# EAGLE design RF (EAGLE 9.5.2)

## Sheet 1 of 3: Board to Board Headers
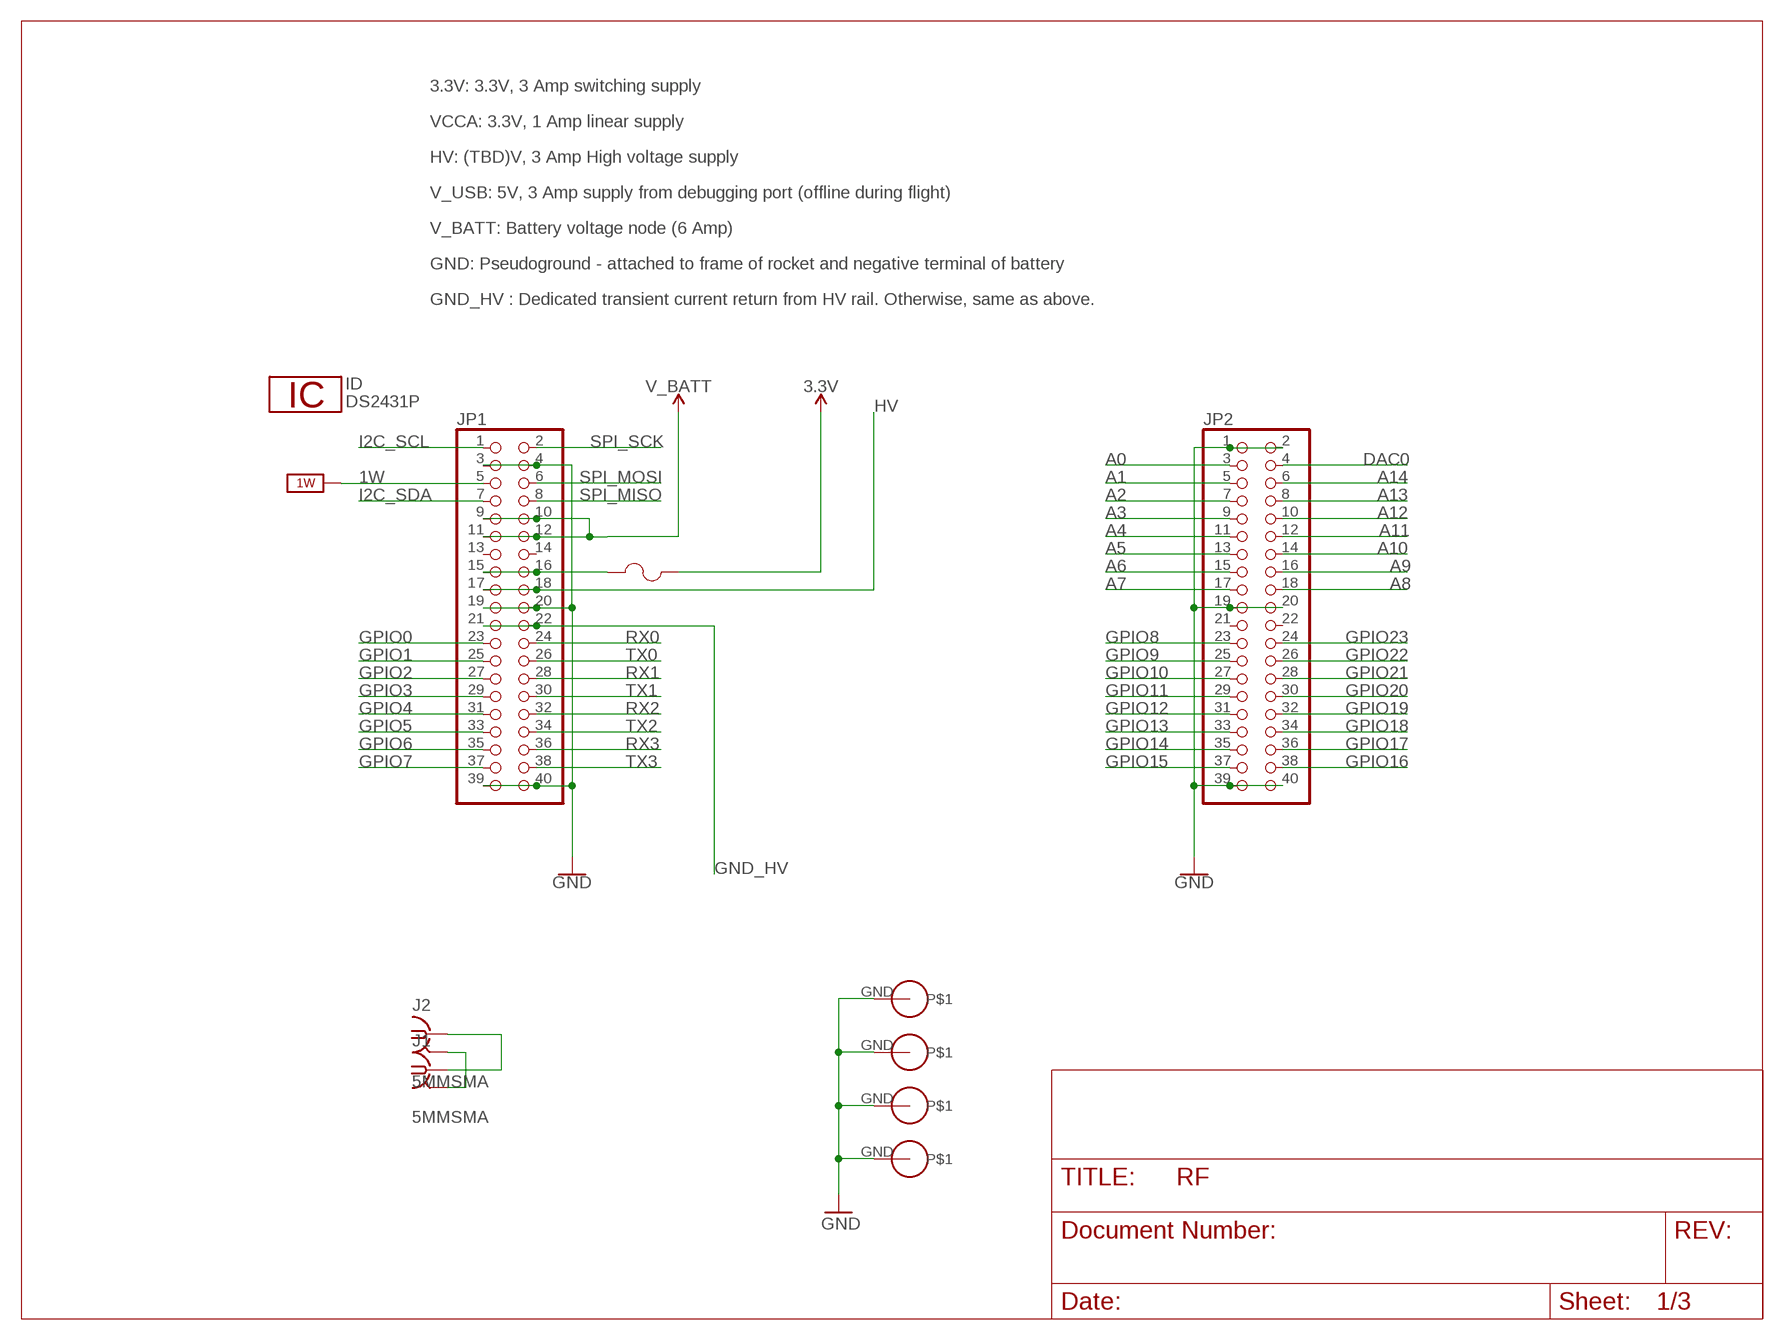
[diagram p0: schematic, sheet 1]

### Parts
F1  0603SFF150F/32-2  [FUS0603_TYCO]
ID  DS2431P  [TSOC6]
J1  5MMSMA  [5MMSMA]
J2  5MMSMA  [5MMSMA]
JP1  PINHD-2X20  [2X20]
JP2  PINHD-2X20  [2X20]
U$1  PS/104-MOUNTING-HOLE  [PC/104-MOUNTING-HOLE]
U$2  PS/104-MOUNTING-HOLE  [PC/104-MOUNTING-HOLE]
U$3  PS/104-MOUNTING-HOLE  [PC/104-MOUNTING-HOLE]
U$4  PS/104-MOUNTING-HOLE  [PC/104-MOUNTING-HOLE]

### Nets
1W: JP1.5 ; supply symbol labelled 1W_SUP
3.3V: F1.2 ; also sheet 2
A0: JP2.3
A1: JP2.5
A2: JP2.7
A3: JP2.9
A4: JP2.11
A5: JP2.13
A6: JP2.15
A7: JP2.17
A8: JP2.18
A9: JP2.16
A10: JP2.14
A11: JP2.12
A12: JP2.10
A13: JP2.8
A14: JP2.6
DAC0: JP2.4
GND: J1.GND J1.GND1 J1.GND2 J1.GND3 J2.GND J2.GND1 J2.GND2 J2.GND3 JP1.3 JP1.4 JP1.19 JP1.20 JP1.39 JP1.40 JP2.1 JP2.2 JP2.19 JP2.20 JP2.39 JP2.40 U$1.GND U$2.GND U$3.GND U$4.GND ; also sheet 2
GND_HV: JP1.21 JP1.22
GPIO0: JP1.23
GPIO1: JP1.25
GPIO2: JP1.27
GPIO3: JP1.29
GPIO4: JP1.31
GPIO5: JP1.33
GPIO6: JP1.35
GPIO7: JP1.37
GPIO8: JP2.23
GPIO9: JP2.25
GPIO10: JP2.27
GPIO11: JP2.29
GPIO12: JP2.31
GPIO13: JP2.33
GPIO14: JP2.35
GPIO15: JP2.37
GPIO16: JP2.38
GPIO17: JP2.36
GPIO18: JP2.34
GPIO19: JP2.32
GPIO20: JP2.30
GPIO21: JP2.28
GPIO22: JP2.26
GPIO23: JP2.24
HV: JP1.17 JP1.18
I2C_SCL: JP1.1
I2C_SDA: JP1.7
N$3: F1.1 JP1.15 JP1.16
N$4: JP1.9 JP1.10 JP1.11 JP1.12
N$8: J1.RF J2.RF
RX0: JP1.24 ; also sheet 2
RX1: JP1.28 ; also sheet 2
RX2: JP1.32 ; also sheet 2
RX3: JP1.36
SPI_MISO: JP1.8
SPI_MOSI: JP1.6
SPI_SCK: JP1.2
TX0: JP1.26 ; also sheet 2
TX1: JP1.30 ; also sheet 2
TX2: JP1.34 ; also sheet 2
TX3: JP1.38
Unconnected: JP1.13 JP1.14 JP2.21 JP2.22

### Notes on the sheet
- 3.3V: 3.3V, 3 Amp switching supply
- VCCA: 3.3V, 1 Amp linear supply
- HV: (TBD)V, 3 Amp High voltage supply
- V_USB: 5V, 3 Amp supply from debugging port (offline during flight)
- V_BATT: Battery voltage node (6 Amp)
- GND: Pseudoground - attached to frame of rocket and negative terminal of battery
- GND_HV : Dedicated transient current return from HV rail. Otherwise, same as above.

## Sheet 2 of 3: RN2483 434MHz RF module
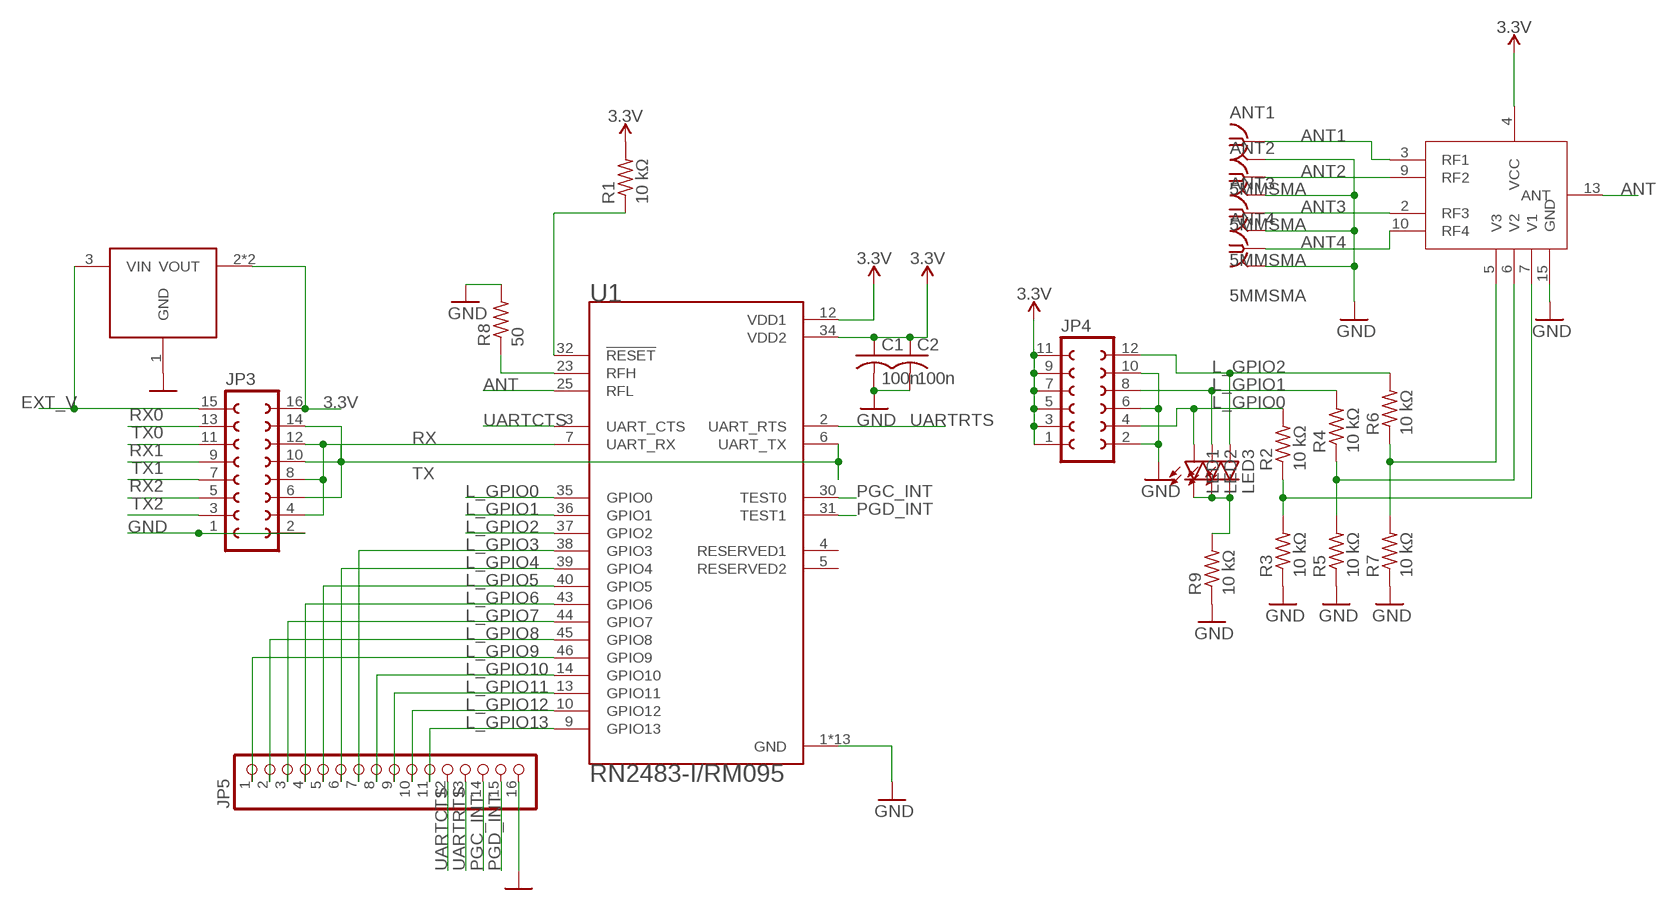
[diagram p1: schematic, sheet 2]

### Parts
ANT1  5MMSMA  [5MMSMA]
ANT2  5MMSMA  [5MMSMA]
ANT3  5MMSMA  [5MMSMA]
ANT4  5MMSMA  [5MMSMA]
C1  100n  C-USC0805  [C0805]
C2  100n  C-USC0805  [C0805]
JP3  FE08-2  [FE08-2]
JP4  FE06-2  [FE06-2]
JP5  PINHD-1X16  [1X16]
LED1  LEDSMT1206  [1206]
LED2  LEDSMT1206  [1206]
LED3  LEDSMT1206  [1206]
R1  10 kΩ  R-US_R1206  [R1206]
R2  10 kΩ  R-US_R1206  [R1206]
R3  10 kΩ  R-US_R1206  [R1206]
R4  10 kΩ  R-US_R1206  [R1206]
R5  10 kΩ  R-US_R1206  [R1206]
R6  10 kΩ  R-US_R1206  [R1206]
R7  10 kΩ  R-US_R1206  [R1206]
R8  50  R-US_R1206  [R1206]
R9  10 kΩ  R-US_R1206  [R1206]
U1  RN2483-I/RM095  [MICROCHIP_RN2483-I/RM095]
U2  SKY13414  [QFN45P200X200X55-15N]
U3  LDL1117S33R  [SOT223]

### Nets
3.3V: C1.1 C2.1 JP3.16 JP4.1 JP4.3 JP4.5 JP4.7 JP4.9 JP4.11 R1.2 U1.12(VDD1) U1.34(VDD2) U2.4(VCC) U3.2(VOUT) U3.4(VOUT) ; also sheet 1
ANT: U1.25(RFL) U2.13(ANT)
ANT1: ANT1.RF U2.3(RF1)
ANT2: ANT2.RF U2.9(RF2)
ANT3: ANT3.RF U2.2(RF3)
ANT4: ANT4.RF U2.10(RF4)
EXT_V: JP3.15 U3.3(VIN)
GND: ANT1.GND ANT1.GND1 ANT1.GND2 ANT1.GND3 ANT2.GND ANT2.GND1 ANT2.GND2 ANT2.GND3 ANT3.GND ANT3.GND1 ANT3.GND2 ANT3.GND3 ANT4.GND ANT4.GND1 ANT4.GND2 ANT4.GND3 C1.2 C2.2 JP3.1 JP3.2 JP4.2 JP4.6 JP4.10 JP5.16 R3.1 R5.1 R7.1 R8.2 R9.1 U1.1(GND) U1.8(GND) U1.11(GND) U1.20(GND) U1.21(GND) U1.22(GND) U1.24(GND) U1.26(GND) U1.27(GND) U1.28(GND) U1.33(GND) U1.41(GND) U1.47(GND) U2.15(GND) U3.1(GND) ; also sheet 1
L_GPIO0: JP4.4 LED1.A R2.2 U1.35(GPIO0)
L_GPIO1: JP4.8 LED2.A R4.2 U1.36(GPIO1)
L_GPIO2: JP4.12 LED3.A R6.2 U1.37(GPIO2)
L_GPIO3: JP5.7 U1.38(GPIO3)
L_GPIO4: JP5.6 U1.39(GPIO4)
L_GPIO5: JP5.5 U1.40(GPIO5)
L_GPIO6: JP5.4 U1.43(GPIO6)
L_GPIO7: JP5.3 U1.44(GPIO7)
L_GPIO8: JP5.2 U1.45(GPIO8)
L_GPIO9: JP5.1 U1.46(GPIO9)
L_GPIO10: JP5.8 U1.14(GPIO10)
L_GPIO11: JP5.9 U1.13(GPIO11)
L_GPIO12: JP5.10 U1.10(GPIO12)
L_GPIO13: JP5.11 U1.9(GPIO13)
N$1: R2.1 R3.2 U2.7(V1)
N$2: R4.1 R5.2 U2.6(V2)
N$5: LED1.C LED2.C LED3.C R9.2
N$7: R6.1 R7.2 U2.5(V3)
N$9: R1.1 U1.32(!RESET)
N$10: R8.1 U1.23(RFH)
PGC_INT: JP5.14 U1.30(TEST0)
PGD_INT: JP5.15 U1.31(TEST1)
RX: JP3.6 JP3.10 JP3.14 U1.6(UART_TX)
RX0: JP3.13 ; also sheet 1
RX1: JP3.9 ; also sheet 1
RX2: JP3.5 ; also sheet 1
TX: JP3.4 JP3.8 JP3.12 U1.7(UART_RX)
TX0: JP3.11 ; also sheet 1
TX1: JP3.7 ; also sheet 1
TX2: JP3.3 ; also sheet 1
UARTCTS: JP5.12 U1.3(UART_CTS)
UARTRTS: JP5.13 U1.2(UART_RTS)
Unconnected: U1.4(RESERVED1) U1.5(RESERVED2)

## Sheet 3 of 3: RN2903 903MHz RF module

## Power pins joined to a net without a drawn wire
1W: ID.2(1W)
GND: ID.1(GND)

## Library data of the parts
ANT1-ANT4 J1 J2 = CUINSPACE_Managed:5MMSMA
C1 C2 = rcl:C-US: CAPACITOR, American symbol; SPICEPREFIX: C
F1 = CU inSpace 2019 Parts:0603SFF150F/32-2; MANUFACTURER_PART_NUMBER: 0603SFF150F322; VENDOR: Littelfuse Inc
ID = 1wire:DS2431: 1024-Bit EEPROM
JP1 JP2 = pinhead:PINHD-2X20: PIN HEADER
JP3 = con-lsta:FE08-2: FEMALE HEADER; OC_FARNELL: unknown; OC_NEWARK: unknown
JP4 = con-lsta:FE06-2: FEMALE HEADER; OC_FARNELL: unknown; OC_NEWARK: unknown
JP5 = pinhead:PINHD-1X16: PIN HEADER
LED1-LED3 = led:LED: LED
R1-R9 = rcl:R-US_: RESISTOR, American symbol; SPICEPREFIX: R
U1 = RN2483-I_RM095:RN2483-I/RM095: Sub-GHz Dual Band Long Range Transceiver LoRa Module; AVAILABILITY: Unavailable; DESCRIPTION: Sub-GHz Dual Band Long Range Transceiver LoRa Module; MF: Microchip; MP: RN2483-I/RM095; PACKAGE: None; PRICE: None
U2 = CUINSPACE_Managed:SKY13414
U3 = CUINSPACE_Managed:LDL1117S33R
U$1-U$4 = CU inSpace 2019 Parts:PS/104-MOUNTING-HOLE: Mounting hole for PC/104 board.

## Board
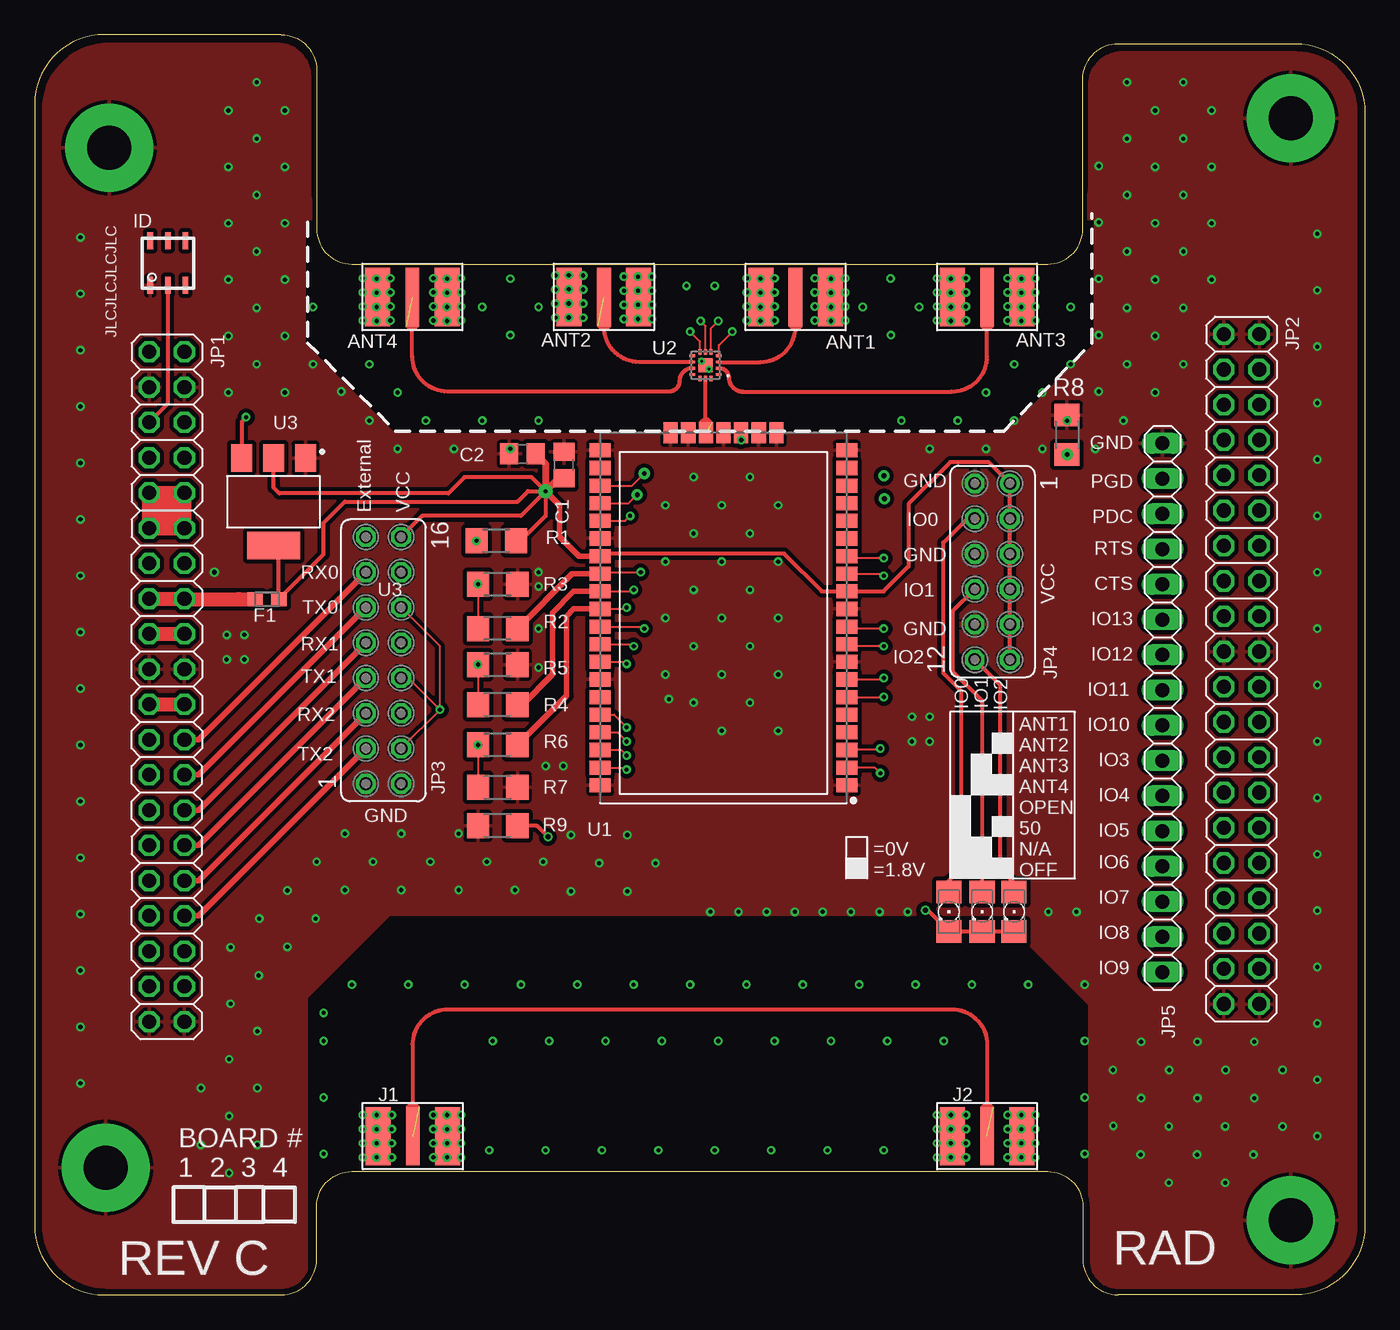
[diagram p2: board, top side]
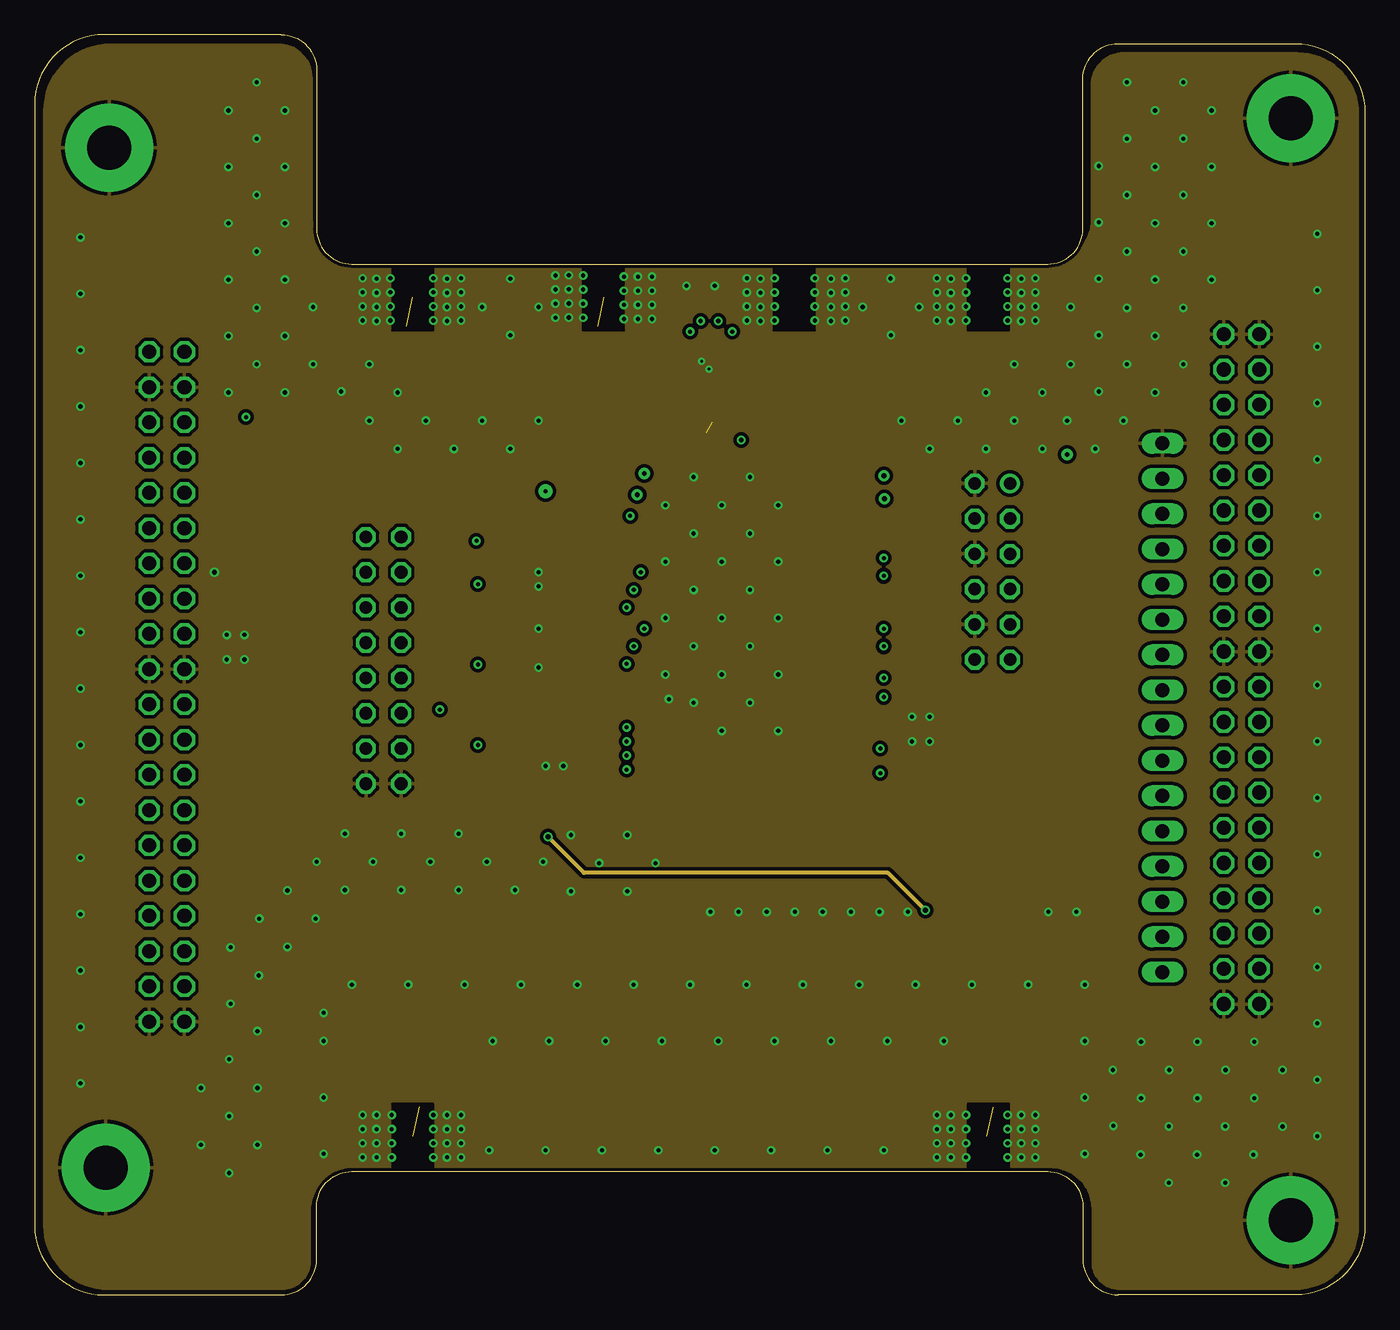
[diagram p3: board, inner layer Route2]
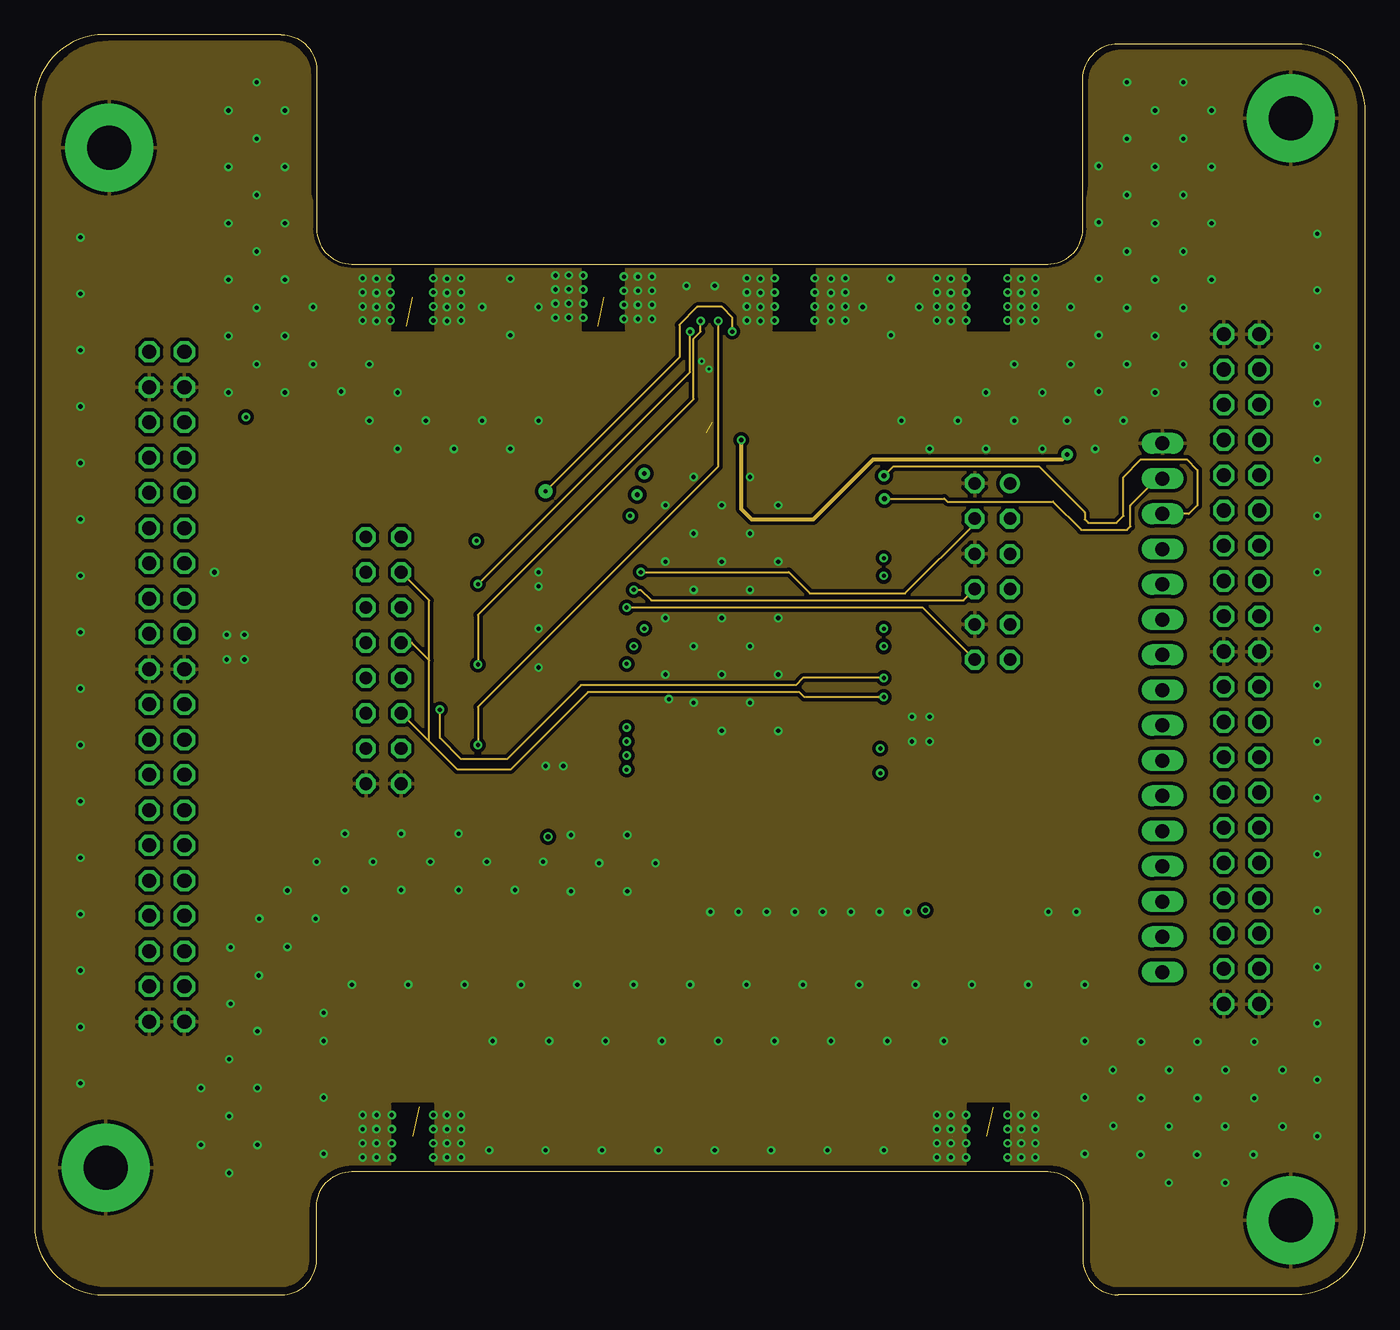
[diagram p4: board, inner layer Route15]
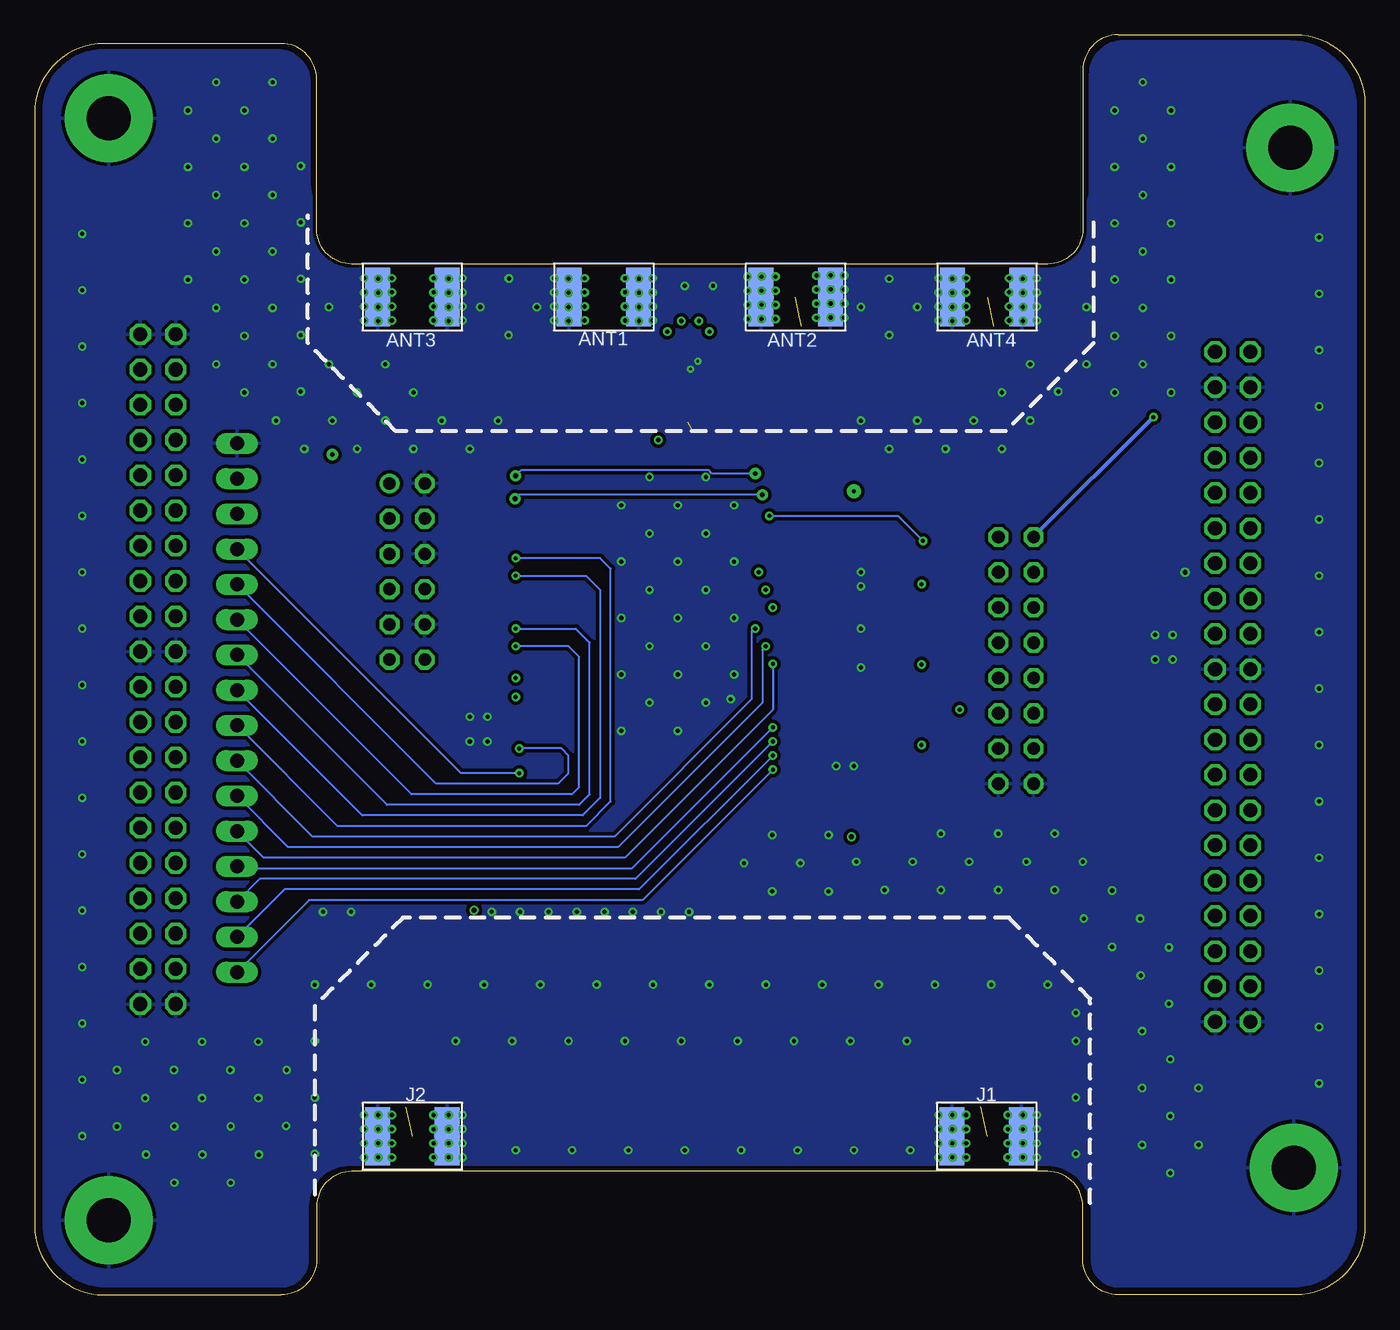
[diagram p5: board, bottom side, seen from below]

Size 95.89 x 90.81 mm. Coordinates in mm from the lower left corner, seen from the top.
Outline: 0,85.81 0,5 arc90 5,0 17.78,0 arc90 20.32,2.54 20.32,6.35 arc-90 22.86,8.89 73.03,8.89 arc-90 75.56,6.35 75.56,2.54 arc90 78.11,0 90.89,0 arc90 95.89,5 95.89,85.17 arc90 90.89,90.17 78.11,90.17 arc90 75.56,87.63 75.56,76.82 arc-90 73.03,74.28 22.86,74.28 arc-90 20.32,76.82 20.32,88.27 arc90 17.78,90.81 5,90.81 arc90 0,85.81
Copper layers (1+2*15+16): Top 0.035mm / dielectric 0.2mm / Route2 0.0175mm / dielectric 1.065mm / Route15 0.0175mm / dielectric 0.2mm / Bottom 0.035mm
Design rules "dirt_cheap_dirty_boards.v1 *": minimum track width 5mil, minimum drill 0.2mm, track to track 5mil, track to pad 5mil, pad to pad 5mil, via to via 5mil, smd to smd 0mil, copper to edge 10mil, drill to drill 10mil, minimum pad ring 10mil, minimum via ring 6mil, stop-mask expansion 2mil, vias tented up to drill 25mil, thermal gap 10mil

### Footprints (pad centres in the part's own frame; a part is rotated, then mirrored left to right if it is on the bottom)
5MMSMA = smd 1.8 x 4.2 bottom: GND 2.5,0; GND2 -2.5,0 | smd 1.8 x 4.2: GND1 -2.5,0; GND3 2.5,0 | smd 1 x 4.2: RF 0,0
C0805 = smd 1.3 x 1.5: 1 -0.95,0; 2 0.95,0
FUS0603_TYCO = smd 1.092 x 0.991: 1 -0.851,0; 2 0.851,0
TSOC6 = smd 0.406 x 1.219: 1 -1.27,-1.6; 2 0,-1.6; 3 1.27,-1.6; 4 1.27,1.6; 5 0,1.6; 6 -1.27,1.6
2X20 = drill 1.016 octagon: 1 -24.13,-1.27; 2 -24.13,1.27; 3 -21.59,-1.27; 4 -21.59,1.27; 5 -19.05,-1.27; 6 -19.05,1.27; 7 -16.51,-1.27; 8 -16.51,1.27; 9 -13.97,-1.27; 10 -13.97,1.27; 11 -11.43,-1.27; 12 -11.43,1.27; 13 -8.89,-1.27; 14 -8.89,1.27; 15 -6.35,-1.27; 16 -6.35,1.27; 17 -3.81,-1.27; 18 -3.81,1.27; 19 -1.27,-1.27; 20 -1.27,1.27; 21 1.27,-1.27; 22 1.27,1.27; 23 3.81,-1.27; 24 3.81,1.27; 25 6.35,-1.27; 26 6.35,1.27; 27 8.89,-1.27; 28 8.89,1.27; 29 11.43,-1.27; 30 11.43,1.27; 31 13.97,-1.27; 32 13.97,1.27; 33 16.51,-1.27; 34 16.51,1.27; 35 19.05,-1.27; 36 19.05,1.27; 37 21.59,-1.27; 38 21.59,1.27; 39 24.13,-1.27; 40 24.13,1.27
FE08-2 = drill 0.914 octagon: 1 -8.89,1.27; 2 -8.89,-1.27; 3 -6.35,1.27; 4 -6.35,-1.27; 5 -3.81,1.27; 6 -3.81,-1.27; 7 -1.27,1.27; 8 -1.27,-1.27; 9 1.27,1.27; 10 1.27,-1.27; 11 3.81,1.27; 12 3.81,-1.27; 13 6.35,1.27; 14 6.35,-1.27; 15 8.89,1.27; 16 8.89,-1.27
FE06-2 = drill 0.914: 1 -6.35,1.27 | drill 0.914 octagon: 2 -6.35,-1.27; 3 -3.81,1.27; 4 -3.81,-1.27; 5 -1.27,1.27; 6 -1.27,-1.27; 7 1.27,1.27; 8 1.27,-1.27; 9 3.81,1.27; 10 3.81,-1.27; 11 6.35,1.27; 12 6.35,-1.27
1X16 = drill 1.016 long: 1 -19.05,0; 2 -16.51,0; 3 -13.97,0; 4 -11.43,0; 5 -8.89,0; 6 -6.35,0; 7 -3.81,0; 8 -1.27,0; 9 1.27,0; 10 3.81,0; 11 6.35,0; 12 8.89,0; 13 11.43,0; 14 13.97,0; 15 16.51,0; 16 19.05,0
1206 = smd 1.6 x 1.803: A -1.422,0; C 1.422,0
R1206 = smd 1.6 x 1.803: 1 -1.422,0; 2 1.422,0
MICROCHIP_RN2483-I/RM095 = smd 1.524 x 1.016: 1 -8.89,12.065; 2 -8.89,10.795; 3 -8.89,9.525; 4 -8.89,8.255; 5 -8.89,6.985; 6 -8.89,5.715; 7 -8.89,4.445; 8 -8.89,3.175; 9 -8.89,1.905; 10 -8.89,0.635; 11 -8.89,-0.635; 12 -8.89,-1.905; 13 -8.89,-3.175; 14 -8.89,-4.445; 15 -8.89,-5.715; 16 -8.89,-6.985; 17 -8.89,-8.255; 18 -8.89,-9.525; 19 -8.89,-10.795; 20 -8.89,-12.065; 28 8.89,-12.065; 29 8.89,-10.795; 30 8.89,-9.525; 31 8.89,-8.255; 32 8.89,-6.985; 33 8.89,-5.715; 34 8.89,-4.445; 35 8.89,-3.175; 36 8.89,-1.905; 37 8.89,-0.635; 38 8.89,0.635; 39 8.89,1.905; 40 8.89,3.175; 41 8.89,4.445; 42 8.89,5.715; 43 8.89,6.985; 44 8.89,8.255; 45 8.89,9.525; 46 8.89,10.795; 47 8.89,12.065 | smd 1.016 x 1.524: 21 -3.81,-13.335; 22 -2.54,-13.335; 23 -1.27,-13.335; 24 0,-13.335; 25 1.27,-13.335; 26 2.54,-13.335; 27 3.81,-13.335
QFN45P200X200X55-15N = smd 0.2 x 0.395: 1 -0.675,-0.953; 2 -0.225,-0.953; 3 0.225,-0.953; 4 0.675,-0.953; 8 0.675,0.953; 9 0.225,0.953; 10 -0.225,0.953; 11 -0.675,0.953 | smd 0.395 x 0.2: 5 0.953,-0.4; 6 0.953,0; 7 0.953,0.4; 12 -0.953,0.4; 13 -0.953,0; 14 -0.953,-0.4 | smd 1 x 1: 15 0,0
SOT223 = smd 1.5 x 2: 1 -2.3,-3.15; 2 0,-3.15; 3 2.3,-3.15 | smd 3.8 x 2: 4 0,3.15
PC/104-MOUNTING-HOLE = drill 3.175 pad 6.35: GND 0,0

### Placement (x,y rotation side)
ANT1  54.85,71.9 180 top
ANT2  41.04,71.9 0 top
ANT3  68.66,71.9 0 top
ANT4  27.22,71.9 0 top
C1  38.15,59.79 90 top
C2  35.15,60.6 180 top
F1  16.75,50.13 0 top
ID  9.6,74.35 0 top
J1  27.26,11.43 0 top
J2  68.66,11.43 0 top
JP1  9.53,43.81 270 top
JP2  87,45.09 270 top
JP3  25.15,45.72 90 top
JP4  69.04,52.12 270 top
JP5  81.3,42.3 90 top
LED1  65.9,27.6 270 top
LED2  68.3,27.6 270 top
LED3  70.6,27.6 270 top
R1  33.27,54.33 0 top
R2  33.38,48.01 0 top
R3  33.38,51.21 180 top
R4  33.38,42.52 0 top
R5  33.38,45.42 180 top
R6  33.38,39.62 0 top
R7  33.38,36.58 180 top
R8  74.42,61.98 90 top
R9  33.38,33.8 0 top
U1  49.65,48.79 180 top
U2  48.36,66.99 90 top
U3  17.22,57.15 180 top
U$1  5.36,82.65 0 top
U$2  90.55,84.79 0 top
U$3  5.13,9.17 0 top
U$4  90.55,5.36 0 top

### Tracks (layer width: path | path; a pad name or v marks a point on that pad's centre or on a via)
1W
  Top 0.305: ID.2 9.6,64.21 JP1.5
3.3V  (via drill 0.3 pad 0.45, 0.3 pad 1)
  Top 0.127: U2.4 49.31,68.43 v50.29,69.41
  Top 0.305: 17.6,53.62 F1.2 20.83,53.35 20.83,55.63 22.35,57.15 34.8,57.15 35.56,57.91 v36.83,57.91 | U3.2 17.22,58.17 17.63,57.76 29.82,57.76 30.99,58.93 35.81,58.93 v36.83,57.91 | v36.83,57.91 35.05,56.13 27.94,56.13 JP3.16 | v36.83,57.91 36.83,56.13 35.11,54.42 34.78,54.42 | U1.34 40.94,53.41 54.03,53.41 56.75,50.69 U1.12 61.19,50.69 63,52.5 63,57 66,60 68.78,60 JP4.1 | JP4.11 JP4.9 JP4.7 JP4.5 JP4.3 JP4.1 | JP4.1 70.65,58.81
  Top 0.406: v36.83,57.91 37.85,56.9 37.85,54.61 39.22,53.23 U1.34 | 34.78,54.42 R1.2
  Top 0.508: C2.1 36.83,59.87 v36.83,57.91 37.76,58.84 C1.1
  Top 1.016: 17.6,53.62 U3.4
  Route15 0.127: v50.29,69.41 50.29,70.42 49.53,71.18 47.75,71.18 46.47,69.9 46.47,67.55 v36.83,57.91
ANT  (1 unrouted)
  Top 0.102: 48.84,62.88 48.54,63.18 48.24,63.18 48.04,62.98 | 48.04,62.98 47.94,62.88 48.24,62.88 48.24,63.08 48.14,62.98 | 48.14,62.98 48.04,62.98 | 48.14,62.98 48.54,62.98 48.54,63.08 48.64,62.98 | 48.64,62.98 48.74,62.88 48.54,62.88 48.64,62.98
  Top 0.293: 48.36,62.14 arc90 U1.25 48.36,62.14 | 48.36,62.14 U2.13
ANT1
  Top 0.102: 54.4,69.8 54.7,69.5 55,69.5 55.2,69.7 | 55.2,69.7 55.3,69.8 55,69.8 55,69.6 55.1,69.7 | 55.1,69.7 55.2,69.7 | 55.1,69.7 54.7,69.7 54.7,69.6 54.6,69.7 | 54.6,69.7 54.5,69.8 54.7,69.8 54.6,69.7
  Top 0.127: ANT1.RF 54.85,69.8 54.7,69.8
  Top 0.293: U2.3 52.31,67.22 arc90 54.85,69.76 ANT1.RF
ANT2  (1 unrouted)
  Top 0.102: 40.6,69.8 40.9,69.5 41.2,69.5 41.4,69.7 | 41.4,69.7 41.5,69.8 41.2,69.8 41.2,69.6 41.3,69.7 | 41.3,69.7 41.4,69.7 | 41.3,69.7 40.9,69.7 40.9,69.6 40.8,69.7 | 40.8,69.7 40.7,69.8 40.9,69.8 40.8,69.7
  Top 0.293: U2.9 43.58,67.22 arc-90 41.04,69.76 ANT2.RF
ANT3
  Top 0.102: 68.2,69.8 68.5,69.5 68.8,69.5 69,69.7 | 69,69.7 69.1,69.8 68.8,69.8 68.8,69.6 68.9,69.7 | 68.9,69.7 69,69.7 | 68.9,69.7 68.5,69.7 68.5,69.6 68.4,69.7 | 68.4,69.7 68.3,69.8 68.5,69.8 68.4,69.7
  Top 0.127: 68.5,69.8 68.66,69.8 68.66,70.5
  Top 0.293: U2.2 49.37,66.77 arc-90 50.04,66.1 arc90 51.05,65.09 66.12,65.09 arc90 68.66,67.63 68.66,70.5 ANT3.RF
ANT4  (1 unrouted)
  Top 0.102: 26.77,69.81 27.07,69.51 27.37,69.51 27.57,69.71 | 27.57,69.71 27.67,69.81 27.37,69.81 27.37,69.61 27.47,69.71 | 27.47,69.71 27.57,69.71 | 27.47,69.71 27.07,69.71 27.07,69.61 26.97,69.71 | 26.97,69.71 26.87,69.81 27.07,69.81 26.97,69.71
  Top 0.293: U2.10 U2.10 arc90 46.48,65.85 arc-90 45.72,65.09 29.76,65.09 arc-90 27.22,67.63 ANT4.RF
EXT_V  (via drill 0.3 pad 0.45)
  Top 0.305: v15.24,63.25 14.92,62.93 U3.3
  Bottom 0.305: JP3.15 v15.24,63.25
GND  (via drill 0.2 pad 0.45, 0.3 pad 0.45, 0.35)  (12 unrouted)
  Top 0.127: U2.15 48.62,66.74 v48.62,66.71
  other vias: 12.95,52.07 24.64,73.22 24.64,72.2 24.64,71.18 24.64,70.17 29.72,73.22 29.72,72.2 29.72,71.18 29.72,70.17 24.13,67.06 68.58,65.02 70.61,67.06 13.97,65.02 16,67.06 18.03,65.02 20.07,67.06 13.97,69.09 16,71.12 18.03,69.09 22.1,65.09 13.97,73.15 16,75.18 18.03,73.15 20.07,71.18 26.16,65.02 13.97,77.22 16,79.25 18.03,77.22 13.97,81.28 16,83.31 18.03,81.28 13.97,85.34 16,87.38 18.03,85.34 32.26,71.18 34.29,73.22 36.32,71.18 61.7,73.24 59.69,71.18 63.75,71.18 80.77,77.22 82.8,79.25 84.84,77.22 80.77,81.28 82.8,83.31 84.84,81.28 80.77,85.34 82.8,87.38 84.84,85.34 80.77,65.02 82.8,67.06 80.77,69.09 82.8,71.12 80.77,73.15 82.8,75.18 84.84,73.15 74.68,67.06 78.74,67.06 76.71,65.09 78.74,71.12 74.68,71.18 76.71,69.15 78.74,75.18 76.71,73.22 78.74,79.25 76.71,77.28 78.74,83.31 76.71,81.34 78.74,87.38 74.42,62.99 76.45,60.96 78.49,62.99 68.58,60.96 70.61,62.99 72.64,60.96 62.48,62.99 64.52,60.96 66.55,62.99 32.26,62.99 24.13,62.99 26.16,60.96 30.23,60.96 28.19,62.99 45.47,56.9 47.5,58.93 49.53,56.9 51.56,58.93 53.59,56.9 45.47,52.83 47.5,54.86 49.53,52.83 51.56,54.86 53.59,52.83 45.47,48.77 47.5,50.8 49.53,48.77 51.56,50.8 53.59,48.77 45.47,44.7 47.5,46.74 49.53,44.7 51.56,46.74 53.59,44.7 45.72,42.93 47.5,42.67 49.53,40.64 51.56,42.67 53.59,40.64 48.08,67.27 22.86,22.35 26.92,22.35 30.99,22.35 35.05,22.35 39.12,22.35 20.83,10.16 20.83,14.22 20.83,20.32 20.83,18.29 33.02,18.29 37.08,18.29 41.15,18.29 45.21,18.29 49.28,18.29 53.34,18.29 57.4,18.29 61.47,18.29 65.53,18.29 75.69,18.29 47.24,22.35 43.18,22.35 51.31,22.35 55.37,22.35 59.44,22.35 63.5,22.35 67.56,22.35 71.63,22.35 75.69,22.35 75.69,14.22 75.69,10.16 40.89,10.41 36.83,10.41 44.96,10.41 49.02,10.41 53.09,10.41 57.15,10.41 61.21,10.41 32.77,10.41 24.64,12.95 24.64,11.94 24.64,10.92 24.64,9.91 29.72,12.95 29.72,11.94 29.72,10.92 29.72,9.91 66.04,12.95 66.04,11.94 66.04,10.92 66.04,9.91 71.12,12.95 71.12,11.94 71.12,10.92 71.12,9.91 38.51,73.47 38.51,72.45 38.51,71.44 38.51,70.42 43.49,73.37 43.49,72.35 43.49,71.34 43.49,70.32 52.32,73.22 52.32,72.2 52.32,71.18 52.32,70.17 57.4,73.22 57.4,72.2 57.4,71.18 57.4,70.17 66.04,73.22 66.04,72.2 66.04,71.18 66.04,70.17 71.12,73.22 71.12,72.2 71.12,71.18 71.12,70.17 36.83,38.1 38.1,38.1 36.32,45.21 36.32,48.01 36.32,51.05 36.32,52.07 72.64,65.02 92.46,48.01 92.46,52.07 92.46,56.13 92.46,64.26 92.46,60.2 92.46,68.33 92.46,72.39 92.46,76.45 92.46,11.43 92.46,15.49 92.46,19.56 92.46,27.69 92.46,23.62 92.46,31.75 92.46,35.81 92.46,39.88 92.46,43.94 64.52,41.66 63.25,41.66 64.52,39.88 63.25,39.88 3.3,15.24 3.3,19.3 3.3,23.37 3.3,31.5 3.3,27.43 3.3,35.56 3.3,39.62 3.3,43.69 3.3,47.75 3.3,51.82 3.3,55.88 3.3,59.94 3.3,68.07 3.3,64.01 3.3,72.14 3.3,76.2 36.32,62.99 34.29,60.96 23.64,73.25 23.64,72.24 23.64,71.22 23.64,70.21 25.64,73.25 25.64,72.24 25.64,71.22 25.64,70.21 28.74,73.25 28.74,72.24 28.74,71.22 28.74,70.21 30.74,73.25 30.74,72.24 30.74,71.22 30.74,70.21 37.54,73.45 37.54,72.44 37.54,71.42 37.54,70.41 39.54,73.45 39.54,72.44 39.54,71.42 39.54,70.41 51.34,73.25 51.34,72.24 51.34,71.22 51.34,70.21 53.34,73.25 53.34,72.24 53.34,71.22 53.34,70.21 56.24,73.25 56.24,72.24 56.24,71.22 56.24,70.21 58.44,73.25 58.44,72.24 58.44,71.22 58.44,70.21 65.04,73.25 65.04,72.24 65.04,71.22 65.04,70.21 67.14,73.25 67.14,72.24 67.14,71.22 67.14,70.21 70.14,73.25 70.14,72.24 70.14,71.22 70.14,70.21 72.14,73.25 72.14,72.24 72.14,71.22 72.14,70.21 42.47,73.37 42.47,72.35 42.47,71.34 42.47,70.32 44.5,73.37 44.5,72.35 44.5,71.34 44.5,70.32 49.02,72.71 46.99,72.71 34.29,69.15 61.72,69.15 23.64,12.95 23.64,11.94 23.64,10.92 23.64,9.91 25.74,12.95 25.74,11.94 25.74,10.92 25.74,9.91 28.74,12.95 28.74,11.94 28.74,10.92 28.74,9.91 30.74,12.95 30.74,11.94 30.74,10.92 30.74,9.91 65.04,12.95 65.04,11.94 65.04,10.92 65.04,9.91 67.14,12.95 67.14,11.94 67.14,10.92 67.14,9.91 70.14,12.95 70.14,11.94 70.14,10.92 70.14,9.91 72.14,12.95 72.14,11.94 72.14,10.92 72.14,9.91 60.91,27.6 62.94,27.6 73.07,27.6 75.1,27.6 56.81,27.6 58.84,27.6 48.71,27.6 50.74,27.6 52.77,27.6 54.8,27.6 44.75,31.1 42.72,29.07 40.69,31.1 42.72,33.14 38.66,29.07 38.66,33.14 36.65,31.2 34.62,29.17 32.59,31.2 30.56,29.17 28.52,31.2 30.56,33.24 26.42,29.17 24.39,31.2 26.42,33.24 22.36,29.17 20.32,31.2 22.36,33.24 20.25,27.1 18.22,25.07 16.19,27.1 18.22,29.14 16.15,23 14.12,20.97 14.12,25.04 16.05,19 14.02,16.97 16.05,14.9 14.02,12.87 11.99,14.9 16.05,10.8 14.02,8.77 11.99,10.8 15.12,47.56 13.85,47.56 15.12,45.78 13.85,45.78 77.76,12.17 85.85,16.2 83.82,14.17 81.79,16.2 83.82,18.24 79.76,14.17 77.72,16.2 79.76,18.24 87.85,10.1 85.82,8.07 83.79,10.1 85.82,12.14 81.76,8.07 79.72,10.1 81.76,12.14 89.95,16.2 87.92,14.17 87.92,18.24 89.96,12.13
  pour Top (isolate 0.305, rank 3): 19.81,87.79 19.81,79.5 arc90 22.41,76.9 73.1,76.9 arc90 76.05,79.85 76.05,87.19 arc-90 78.4,89.53 90.92,89.53 arc-90 95.25,85.21 95.25,5.04 arc-90 90.72,0.51 78.11,0.51 arc-90 76.2,2.41 76.2,6.25 arc90 73.18,9.27 22.91,9.27 arc90 19.68,6.05 19.68,2.45 arc-90 17.74,0.51 5.19,0.51 arc-90 0.64,5.06 0.64,85.4 arc-90 5.4,90.17 17.43,90.17 arc-90
  pour Bottom (isolate 0.254): 19.81,87.92 19.81,79.63 arc90 22.41,77.03 73.1,77.03 arc90 76.05,79.98 76.05,87.31 arc-90 78.4,89.66 90.92,89.66 arc-90 95.25,85.33 95.25,5.17 arc-90 90.72,0.64 78.11,0.64 arc-90 76.2,2.54 76.2,6.38 arc90 73.18,9.4 22.91,9.4 arc90 19.68,6.17 19.68,2.58 arc-90 17.74,0.64 5.19,0.64 arc-90 0.64,5.19 0.64,85.53 arc-90 5.4,90.3 17.43,90.3 arc-90
  pour Route15 (isolate 0.254): 19.81,87.92 19.81,79.63 arc90 22.41,77.03 73.1,77.03 arc90 76.05,79.98 76.05,87.31 arc-90 78.4,89.66 90.92,89.66 arc-90 95.25,85.33 95.25,5.17 arc-90 90.72,0.64 78.11,0.64 arc-90 76.2,2.54 76.2,6.38 arc90 73.18,9.4 22.91,9.4 arc90 19.68,6.17 19.68,2.58 arc-90 17.74,0.64 5.19,0.64 arc-90 0.64,5.19 0.64,85.53 arc-90 5.4,90.3 17.43,90.3 arc-90
  pour Route2 (isolate 0.254): 19.91,87.72 19.91,77.93 arc90 23.71,74.13 72.8,74.13 arc90 76.25,77.58 76.25,87.21 arc-90 78.5,89.46 91.02,89.46 arc-90 95.35,85.13 95.35,4.97 arc-90 90.82,0.43 78.2,0.43 arc-90 76.3,2.34 76.3,6.18 arc90 73.28,9.2 23.01,9.2 arc90 19.79,5.97 19.79,2.38 arc-90 17.84,0.43 5.29,0.43 arc-90 0.73,4.99 0.73,85.33 arc-90 5.5,90.1 17.53,90.1 arc-90
  cutout Route15: 25.75,74.25 25.75,69.5 28.75,69.5 28.75,74.25
GND1
  cutout Route2: 25.75,74.25 25.75,69.5 28.75,69.5 28.75,74.25
GND2
  cutout Bottom: 25.75,74.25 25.75,69.5 28.75,69.5 28.75,74.25
GND6
  cutout Route15: 39.5,74.25 39.5,69.5 42.5,69.5 42.5,74.25
GND7
  cutout Route2: 39.5,74.25 39.5,69.5 42.5,69.5 42.5,74.25
GND8
  cutout Bottom: 39.5,74.25 39.5,69.5 42.5,69.5 42.5,74.25
GND9
  cutout Route15: 53.25,74.25 53.25,69.5 56.25,69.5 56.25,74.25
GND10
  cutout Route2: 53.25,74.25 53.25,69.5 56.25,69.5 56.25,74.25
GND11
  cutout Bottom: 53.25,74.25 53.25,69.5 56.25,69.5 56.25,74.25
GND12
  cutout Route15: 67.25,74.25 67.25,69.5 70.25,69.5 70.25,74.25
GND13
  cutout Route2: 67.25,74.25 67.25,69.5 70.25,69.5 70.25,74.25
GND14
  cutout Bottom: 67.25,74.25 67.25,69.5 70.25,69.5 70.25,74.25
GND15
  cutout Route15: 67.25,13.75 67.25,9 70.25,9 70.25,13.75
GND16
  cutout Route2: 67.25,13.75 67.25,9 70.25,9 70.25,13.75
GND17
  cutout Bottom: 67.25,13.75 67.25,9 70.25,9 70.25,13.75
GND18
  cutout Route15: 25.75,13.75 25.75,9 28.75,9 28.75,13.75
GND19
  cutout Route2: 25.75,13.75 25.75,9 28.75,9 28.75,13.75
GND20
  cutout Bottom: 25.75,13.75 25.75,9 28.75,9 28.75,13.75
GND_HV
  Top 1.016: JP1.21 JP1.22
HV
  Top 1.016: JP1.17 JP1.18
KEEPOUT
  cutout Top (no thermals): 19.68,77.28 19.68,68.58 26.04,62.23 69.85,62.23 76.2,68.58 76.2,77.28 75.56,77.28
KEEPOUT1
  cutout Top (no thermals): 75.82,-0.64 75.82,20.83 69.47,27.18 25.65,27.18 19.81,21.34 19.81,-0.64
L_GPIO0  (via drill 0.3 pad 0.45)
  Top 0.127: U1.35 40.87,52.07 v43.69,52.07
  Top 0.305: LED1.A 65.9,29.82 66.8,30.72 66.8,43.5 65.5,44.8 65.5,54.2 67.23,55.93 JP4.4
  Top 0.406: R2.2 38.75,51.96 U1.35
  Route15 0.127: v43.69,52.07 54.36,52.07 55.88,50.55 62.74,50.55 67.77,55.58 JP4.4
L_GPIO1  (via drill 0.3 pad 0.45)
  Top 0.127: U1.36 43.07,50.69 v43.18,50.8
  Top 0.305: JP4.8 66.2,49.28 66.2,44.9 68.3,42.8 LED2.A
  Top 0.406: U1.36 38.86,50.69 37.34,49.17 37.34,44.7 35.15,42.52 R4.2
  Route15 0.127: v43.18,50.8 43.69,50.8 44.45,50.04 66.95,50.04 JP4.8
L_GPIO2  (via drill 0.3 pad 0.45)
  Top 0.127: U1.37 42.56,49.42 v42.67,49.53
  Top 0.305: LED3.A 70.6,29.7 69.6,30.7 69.6,43.94 JP4.12
  Top 0.406: U1.37 38.86,49.42 38.35,48.91 38.35,43.18 R6.2
  Route15 0.127: JP4.12 64.01,49.53 v42.67,49.53
L_GPIO3  (via drill 0.3 pad 0.45)
  Top 0.127: U1.38 43.8,48.15 v43.94,48.01
  Bottom 0.127: v43.94,48.01 44.2,47.75 44.2,42.93 54.1,33.02 75.83,33.02 JP5.7
L_GPIO4  (via drill 0.3 pad 0.45)
  Top 0.127: U1.39 43.03,46.88 v43.18,46.74
  Bottom 0.127: v43.18,46.74 43.43,46.48 43.43,42.67 53.85,32.26 77.61,32.26 JP5.6
L_GPIO5  (via drill 0.3 pad 0.45)
  Top 0.127: U1.40 42.53,45.61 v42.67,45.47
  Bottom 0.127: v42.67,45.47 42.67,42.16 53.34,31.5 79.39,31.5 JP5.5
L_GPIO6  (via drill 0.3 pad 0.45)
  Top 0.127: U1.43 41.76,41.8 v42.67,40.89
  Bottom 0.127: v42.67,40.89 52.83,30.73 81.16,30.73 JP5.4
L_GPIO7  (via drill 0.3 pad 0.45)
  Top 0.127: U1.44 42.02,40.53 v42.67,39.88
  Bottom 0.127: v42.67,39.88 52.58,29.97 79.66,29.97 JP5.3
L_GPIO8  (via drill 0.3 pad 0.45)
  Top 0.127: U1.45 42.27,39.26 v42.67,38.86
  Bottom 0.127: v42.67,38.86 52.32,29.21 77.88,29.21 JP5.2
L_GPIO9  (via drill 0.3 pad 0.45)
  Top 0.127: U1.46 42.53,37.99 v42.67,37.85
  Bottom 0.127: v42.67,37.85 52.07,28.45 76.1,28.45 JP5.1
L_GPIO10  (via drill 0.3 pad 0.45)
  Top 0.127: v61.21,53.09 58.69,53.09 U1.14
  Bottom 0.127: v61.21,53.09 55.12,53.09 54.36,52.32 54.36,35.56 56.13,33.78 74.05,33.78 JP5.8
L_GPIO11  (via drill 0.3 pad 0.45)
  Top 0.127: U1.13 61.07,51.96 v61.21,51.82
  Bottom 0.127: v61.21,51.82 56.13,51.82 55.12,50.8 55.12,35.81 56.39,34.54 72.27,34.54 JP5.9
L_GPIO12  (via drill 0.3 pad 0.45)
  Top 0.127: v61.21,48.01 58.69,48.01 U1.10
  Bottom 0.127: v61.21,48.01 56.9,48.01 55.88,46.99 55.88,36.07 56.64,35.31 70.5,35.31 JP5.10
L_GPIO13  (via drill 0.3 pad 0.45)
  Top 0.127: v61.21,46.74 58.69,46.74 U1.9
  Bottom 0.127: v61.21,46.74 57.4,46.74 56.64,45.97 56.64,36.58 57.15,36.07 68.72,36.07 JP5.11
N$1  (via drill 0.3 pad 0.45)
  Top 0.127: U2.7 47.96,68.69 v47.24,69.41 | R3.2 R2.1
  Route15 0.127: R3.2 47.24,66.5 v47.24,69.41
  other vias: 31.95,51.21
N$2  (via drill 0.3 pad 0.45)
  Top 0.127: U2.6 48.36,69.81 v48.01,70.17 | R5.2 R4.1
  Route15 0.127: R5.2 31.95,49 47.5,64.55 47.5,68.9 48.01,69.41 v48.01,70.17
  other vias: 31.95,45.42
N$3
  Top 1.016: JP1.15 JP1.16 10.79,50.13 14.73,50.13 F1.1
N$4
  Top 1.016: 9,55.24 JP1.11 JP1.9 | 9,55.24 10,55.24 | 10,55.24 JP1.12 JP1.10 10,57.78 | JP1.9 10,57.78 | JP1.9 9,57.78 9,55.24 | 10,55.24 10,57.78
N$5  (via drill 0.35)
  Top 0.305: LED3.C LED2.C LED1.C 64.38,27.7 v64.2,27.7 | v37,33 36.2,33.8 R9.2
  Route2 0.305: v64.2,27.7 61.5,30.4 39.6,30.4 v37,33
N$7  (via drill 0.3 pad 0.45)
  Top 0.127: U2.5 48.76,69.65 v49.28,70.17 | R6.1 R7.2
  Route15 0.127: R6.1 31.95,42.37 49.28,59.69 v49.28,70.17
  other vias: 31.95,39.62
N$8  (2 unrouted)
  Top 0.102: 27.71,13.55 27.41,13.85 27.11,13.85 26.91,13.65 | 26.91,13.65 26.81,13.55 27.11,13.55 27.11,13.75 27.01,13.65 | 27.01,13.65 26.91,13.65 | 27.01,13.65 27.41,13.65 27.41,13.75 27.51,13.65 | 27.51,13.65 27.61,13.55 27.41,13.55 27.51,13.65 | 69.11,13.53 68.81,13.83 68.51,13.83 68.31,13.63 | 68.31,13.63 68.21,13.53 68.51,13.53 68.51,13.73 68.41,13.63 | 68.41,13.63 68.31,13.63 | 68.41,13.63 68.81,13.63 68.81,13.73 68.91,13.63 | 68.91,13.63 69.01,13.53 68.81,13.53 68.91,13.63
  Top 0.293: J1.RF 27.26,18.03 arc-90 29.8,20.57 66.12,20.57 arc-90 68.66,18.03 J2.RF
N$9  (via drill 0.3 pad 0.45)
  Top 0.127: U1.32 42.16,55.77 42.56,55.77 v42.93,56.13
  Bottom 0.127: v42.93,56.13 33.66,56.13 R1.1
  other vias: 31.85,54.33
N$10  (via drill 0.3 pad 0.45, 0.35 pad 0.8)
  Top 0.293: U1.23 v50.92,61.6 v50.93,61.59
  Route15 0.293: v50.93,61.59 50.93,56.64 51.69,55.88 56.13,55.88 60.45,60.2 74.07,60.2 R8.1
  other vias: 74.42,60.55
PGC_INT  (via drill 0.35 pad 0.8)
  Top 0.127: U1.30 43.07,58.31 v43.94,59.18
  Route15 0.127: v61.21,59.02 61.89,59.69 72.39,59.69 75.69,56.39 75.69,55.88 75.95,55.63 77.98,55.63 78.49,56.13 78.49,58.93 79.76,60.2 83.06,60.2 83.82,59.44 83.82,56.9 83.19,56.27 JP5.14
  Bottom 0.127: v43.94,59.18 47.05,59.18 47.29,59.42 60.81,59.42 v61.21,59.02
PGD_INT  (via drill 0.35 pad 0.8)
  Top 0.127: U1.31 42.82,57.04 v43.43,57.66
  Route15 0.127: v61.25,57.37 65.56,57.37 65.79,57.15 73.41,57.15 75.44,55.12 78.74,55.12 78.99,55.37 78.99,56.9 80.91,58.81 JP5.15
  Bottom 0.127: v43.43,57.66 60.96,57.66 v61.25,57.37
RX  (via drill 0.3 pad 0.45)
  Top 0.127: U1.6 v61.21,43.07
  Route15 0.127: v61.21,43.07 55.48,43.07 55.12,43.43 39.88,43.43 34.29,37.85 30.48,37.85 28.45,39.88 | 28.45,39.88 JP3.6 | 28.45,39.88 28.45,45.72 | 28.45,45.72 27.18,46.99 JP3.10 | 28.45,45.72 28.45,50.04 JP3.14
RX0
  Top 0.406: JP3.13 11.81,40.01 JP1.24
RX1
  Top 0.406: JP3.9 11.81,34.92 JP1.28
RX2
  Top 0.406: JP3.5 11.81,29.84 JP1.32
TX  (via drill 0.3 pad 0.45)
  Top 0.127: U1.7 61.11,44.34 v61.21,44.45 | v29.21,42.16 JP3.4 | v29.21,42.16 26.92,44.45 JP3.8 | v29.21,42.16 29.21,46.74 JP3.12
  Route15 0.127: v29.21,42.16 29.21,40.13 30.73,38.61 34.04,38.61 39.37,43.94 54.86,43.94 55.37,44.45 v61.21,44.45
TX0
  Top 0.406: JP3.11 11.81,37.47 JP1.26
TX1
  Top 0.406: JP3.7 11.81,32.38 JP1.30
TX2
  Top 0.406: JP3.3 11.81,27.3 JP1.34
UARTCTS  (via drill 0.3 pad 0.45)
  Top 0.127: v60.96,39.37 60.85,39.26 U1.3
  Bottom 0.127: v60.96,39.37 57.91,39.37 57.4,38.86 57.4,37.59 58.17,36.83 66.94,36.83 JP5.12
UARTRTS  (via drill 0.3 pad 0.45)
  Top 0.127: v60.96,37.59 60.56,37.99 U1.2
  Bottom 0.127: JP5.13 65.16,37.59 v60.96,37.59

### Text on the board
tPlace: JLCJLCJLCJLC | BOARD # / 1 2 3 4 | RAD | REV C
tNames: U3 | GND | PGD | GND | PDC | External | VCC | IO0 | RTS | GND | RX0 | CTS | IO1 | VCC | TX0 | IO13 | GND | IO12 | RX1 | IO2 | TX1 | IO11 | IO0 | IO1 | IO2 | IO10 | RX2 | ANT1 | ANT2 | IO3 | TX2 | ANT3 | IO4 | ANT4 | OPEN | GND | IO5 | 50 | =0V | N/A | IO6 | =1.8V | OFF | IO7 | IO8 | IO9 | JP5

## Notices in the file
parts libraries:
SparkFun-PowerSymbols: Licensing: Creative Commons ShareAlike 4.0 International - https://creativecommons.org/licenses/by-sa/4.0
